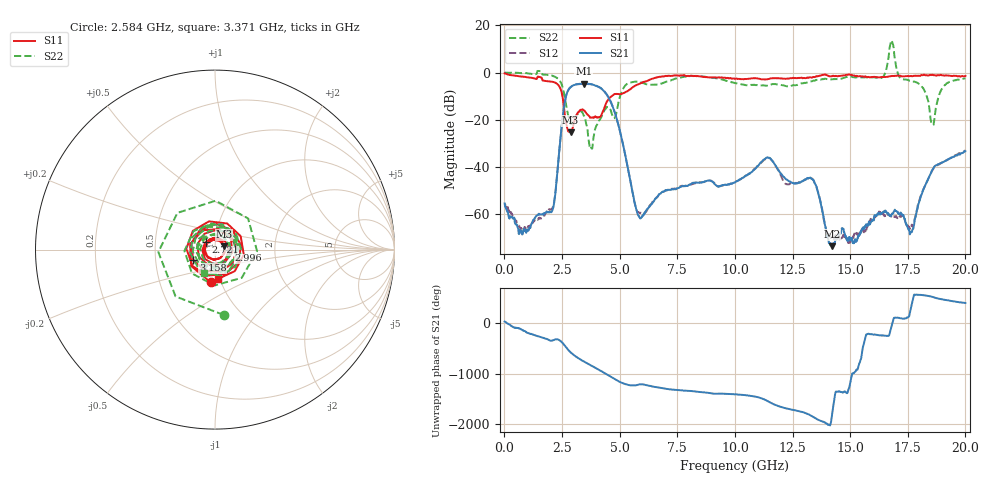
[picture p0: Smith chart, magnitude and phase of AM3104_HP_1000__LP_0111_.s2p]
!Created with skrf (http://scikit-rf.org).
# Hz S RI R 50.0
!freq ReS11 ImS11 ReS21 ImS21 ReS12 ImS12 ReS22 ImS22
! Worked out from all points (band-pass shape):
!   1601 points, 10 MHz to 20 GHz, reference 50 ohm
!   highest |S21| = -4.70 dB at 3.446 GHz (marker M1); lowest = -73.8 dB at 14.22 GHz (marker M2)
!   |S21| within 3 dB of the highest: 2.759 GHz to 4.308 GHz (1.549 GHz wide, 43.8 % of centre)
!   lowest |S11| = -25.4 dB at 2.871 GHz (marker M3), VSWR 1.11, Z = 55.3 + j2.07 ohm
!   |S11| at or under -10 dB: 2.518 GHz to 4.656 GHz (2.138 GHz wide, 59.6 % of centre)
!   |S22| runs from -32.4 to 13.6 dB; largest |S21 - S12| = 0.037
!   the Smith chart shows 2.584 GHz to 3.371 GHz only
!   S11 on the Smith chart (normalised r, x): 2.584 GHz: 0.89, -0.33; 2.721 GHz: 0.90, +0.08; 2.996 GHz: 1.17, -0.01; 3.158 GHz: 0.78, -0.09; 3.371 GHz: 0.98, -0.33
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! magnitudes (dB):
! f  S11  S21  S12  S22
! 10 MHz  -0.3  -55.6  -56.1  0.0
! 709.6 MHz  -1.7  -67.1  -66.1  -0.2
! 2.046 GHz  -3.9  -59.3  -58.0  -1.2
! 2.584 GHz  -14.8  -14.8  -14.8  -8.7
! 2.721 GHz  -23.4  -8.6  -8.5  -16.0
! 2.871 GHz  -25.4  -6.2  -6.3  -21.7
! 2.996 GHz  -22.3  -5.4  -5.4  -20.8
! 3.158 GHz  -17.4  -5.0  -5.0  -18.1
! 3.346 GHz  -15.8  -4.8  -4.8  -16.6
! 3.371 GHz  -15.7  -4.8  -4.8  -16.7
! 3.446 GHz  -16.1  -4.7  -4.7  -18.4
! 3.758 GHz  -19.1  -5.0  -5.0  -32.0
! 4.67 GHz  -9.9  -13.7  -13.8  -17.8
! 5.845 GHz  -4.9  -61.1  -59.5  -4.0
! 6.682 GHz  -1.9  -52.2  -52.1  -5.0
! 10.01 GHz  -2.7  -46.7  -46.6  -4.5
! 13.34 GHz  -2.1  -45.2  -45.0  -3.7
! 14.22 GHz  -1.6  -73.8  -70.6  -2.9
! 16.68 GHz  -1.6  -60.4  -60.7  7.2
! 17.66 GHz  -1.6  -67.7  -64.8  -3.8
! 18.56 GHz  -0.9  -41.3  -41.6  -21.8
! 20 GHz  -1.5  -33.5  -33.2  -2.5
